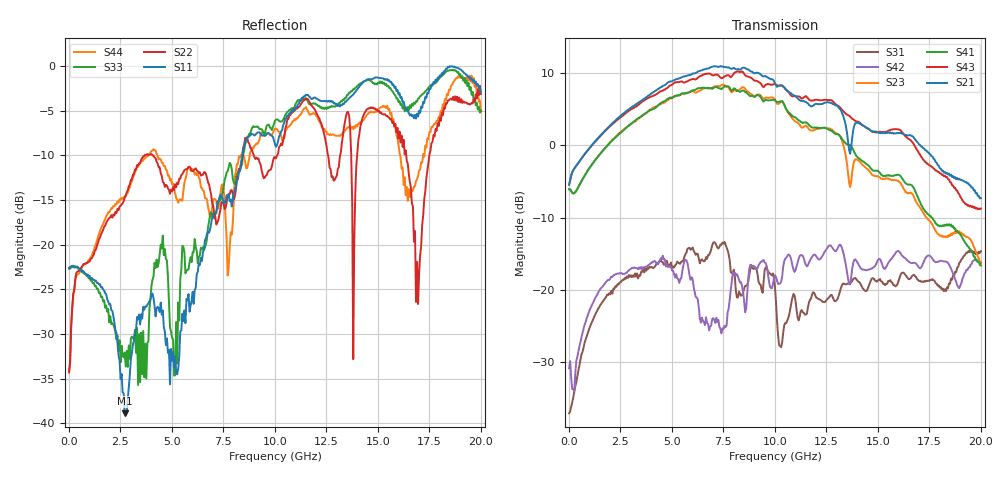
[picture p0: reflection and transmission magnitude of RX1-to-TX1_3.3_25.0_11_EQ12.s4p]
!Agilent Technologies,N5225A,MY51451112,A.09.50.13
!Agilent N5225A: A.09.50.13
!Date: Wednesday, January 31, 2018 11:05:30
!Correction: S11(Full 4 Port(1,2,3,4))
!S12(Full 4 Port(1,2,3,4))
!S13(Full 4 Port(1,2,3,4))
!S14(Full 4 Port(1,2,3,4))
!S21(Full 4 Port(1,2,3,4))
!S22(Full 4 Port(1,2,3,4))
!S23(Full 4 Port(1,2,3,4))
!S24(Full 4 Port(1,2,3,4))
!S31(Full 4 Port(1,2,3,4))
!S32(Full 4 Port(1,2,3,4))
!S33(Full 4 Port(1,2,3,4))
!S34(Full 4 Port(1,2,3,4))
!S41(Full 4 Port(1,2,3,4))
!S42(Full 4 Port(1,2,3,4))
!S43(Full 4 Port(1,2,3,4))
!S44(Full 4 Port(1,2,3,4))
!S4P File: Measurements: <S11,S12,S13,S14>,
!<S21,S22,S23,S24>,
!<S31,S32,S33,S34>,
!<S41,S42,S43,S44>:
# Hz S  RI  R 50
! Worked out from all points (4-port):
!   401 points, 10 MHz to 20 GHz, reference 50 ohm
!   strongest paths, dB at 10 MHz, 5.008 GHz, 10.01 GHz, 15 GHz, 20 GHz:
!     S21: -5.4, 8.9, 8.6, 1.8, -7.3
!     S43: -5.5, 8.4, 8.5, 1.9, -8.7
!     S41: -6.1, 6.6, 6.2, -3.5, -16.6
!     S23: -6.1, 6.5, 6.3, -4.3, -16.3
!     S42: -30.8, -17.3, -18.0, -15.8, -16.2
!     S31: -37.0, -17.1, -19.6, -18.6, -14.6
!   lowest |S11| = -38.9 dB at 2.709 GHz (marker M1), VSWR 1.02, Z = 49.1 - j0.692 ohm
!   |S11| at or under -10 dB: start of sweep to 8.419 GHz
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1e7  -0.0742 -0.00323  0.000166 0.000122  0.0141 0.000319  -0.000411 0.000434
     0.5361 0.0133  -0.0132 0.014  -0.498 -0.00158  0.0262 0.0118
     0.0141 0.000738  0.000561 0.000495  -0.0732 -0.00419  -0.00013 0.000555
     -0.4975 -0.000954  0.0263 0.0119  0.5334 0.0126  -0.0129 0.0147
2.70865e9  -0.00891 -0.00705  0.0158 0.00341  0.0515 0.1092  0.0175 0.000763
           1.405 -0.9385  0.1823 0.0166  -1.043 0.7875  0.0999 0.0922
           0.0576 0.1063  0.0189 0.00397  0.00619 0.0241  0.021 0.000796
           -0.9169 0.9124  0.0883 0.0949  1.146 -1.184  0.1833 -0.0338
6.956525e9  -0.034 0.1378  0.0131 -0.0153  0.1406 0.0652  0.0103 -0.0269
            -3.478 0.2448  0.1048 -0.1346  2.426 -0.5749  0.027 0.0291
            0.1512 0.1362  0.0201 -0.0137  0.0266 0.146  0.0232 -0.0303
            1.953 -1.493  0.0628 -0.00685  -2.555 1.683  0.0888 -0.1369
8.6057e9  -0.00279 0.3842  0.000138 -0.00911  0.0669 0.0472  -0.00573 -0.0183
          -0.812 3.293  -0.1197 0.3717  0.1212 -2.4  -0.0143 0.1266
          0.0926 0.0538  0.00919 -0.0168  0.0251 0.3773  -0.00929 -0.0336
          -0.9426 -2.117  -0.0188 0.0719  0.9257 2.862  0.2089 0.1671
1.045478e10  0.1346 0.463  -0.0277 -0.0409  0.0041 0.00676  -0.0545 -0.0121
             2.16 1.293  0.271 0.2898  -1.85 -0.5112  0.0316 0.1822
             -0.0414 0.0393  -0.0351 -0.0386  0.2194 0.4637  -0.0594 -0.0176
             -1.837 0.5087  0.0723 0.1417  2.505 -0.163  0.3949 -0.1036
1.42029e10  0.6695 0.4193  -0.0286 0.000358  0.00706 0.0954  -0.0124 0.0128
            0.2365 -1.368  0.4561 0.1533  0.1213 0.7365  0.1506 0.0352
            0.0195 0.1052  -0.0135 -0.00157  0.7603 0.266  -0.0229 0.0173
            0.6886 0.3814  0.1275 0.0572  -1.142 -0.8067  -0.149 -0.4624
2e10  0.7115 0.0714  0.023 0.0349  -0.0799 0.1593  0.0348 0.0209
      0.0439 0.4295  0.6935 0.0747  -0.0106 -0.1519  0.155 0.0396
      -0.0787 0.168  0.00621 0.0478  0.5633 -0.0238  0.0475 0.0205
      -0.1433 -0.036  0.1484 0.0457  0.3533 0.097  -0.1516 -0.5317
